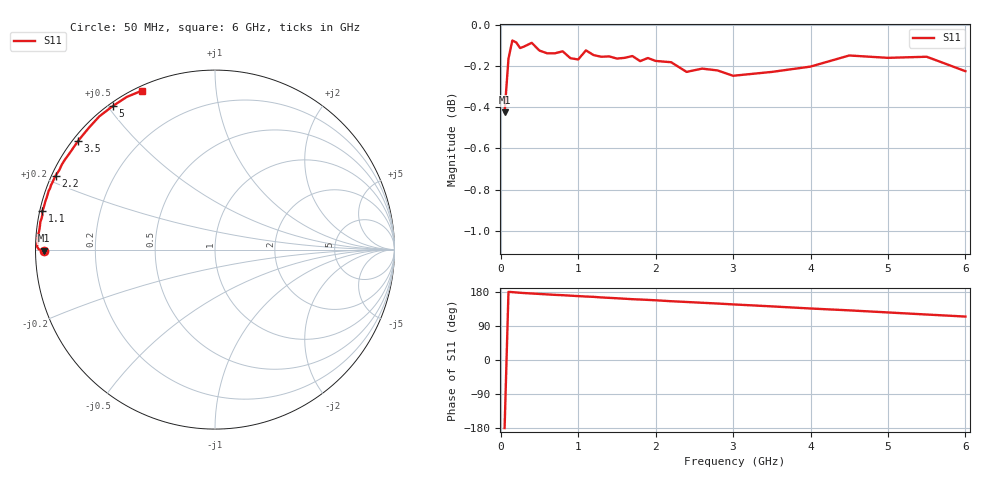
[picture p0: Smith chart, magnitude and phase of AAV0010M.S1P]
! Infineon Technologies  Discrete & RF Semiconductors
! BBY66-02W
! Si Tuning Diode in SCD-80
! VR =
! S-Parameters:  June  2000
# GHz  S  MA  R  50
!  f  S11
! GHz  MAG  ANG
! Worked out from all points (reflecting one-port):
!   34 points, 50 MHz to 6 GHz, reference 50 ohm
!   lowest |S11| = -0.4 dB at 50 MHz (marker M1), VSWR 41.02, Z = 1.22 - j0.174 ohm
!   phase of S11 starts at -180 deg and turns -66 deg over the sweep
!   S11 on the Smith chart (normalised r, x): 50 MHz: 0.02, -0.00; 1.1 GHz: 0.01, +0.11; 2.2 GHz: 0.01, +0.22; 3.5 GHz: 0.01, +0.35; 5 GHz: 0.01, +0.51; 6 GHz: 0.02, +0.64
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0.05  0.9524 -179.6
0.1  0.9814 179.9
0.15  0.9914 179.1
0.25  0.9872 177.4
0.3  0.988 176.7
0.4  0.9901 175.5
0.5  0.9858 174.3
0.7  0.9843 171.9
0.8  0.9854 171.0
1  0.9809 168.6
1.1  0.9859 167.5
1.2  0.9833 166.6
1.3  0.9824 165.1
1.6  0.9818 161.7
1.7  0.9828 160.5
1.8  0.98 159.6
2  0.9801 157.6
2.2  0.9794 155.1
2.4  0.9741 153.1
2.6  0.9759 151.0
2.8  0.9749 149.0
3  0.972 146.7
3.5  0.9741 141.5
4  0.977 135.9
4.5  0.9831 131.0
5  0.9818 125.5
5.5  0.9824 120.0
6  0.9745 114.6
